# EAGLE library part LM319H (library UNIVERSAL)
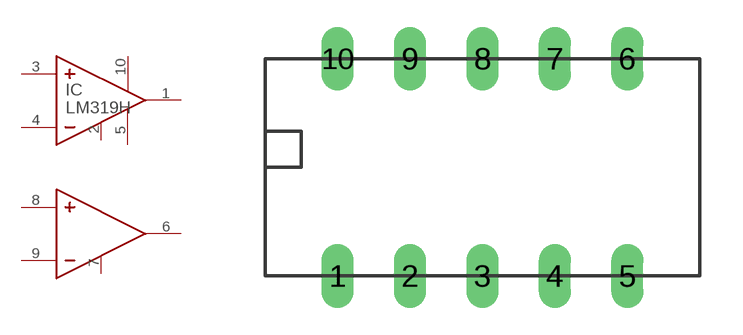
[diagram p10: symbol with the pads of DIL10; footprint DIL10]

Designator prefix IC

## LM319H  [DIL10]
1  1
2  2
3  3
4  4
5  5
6  6
7  7
8  8
9  9
10  10

## Footprint DIL10 (pad centres in mm)
drill 0.61 pad 1.092 long: 1 0,0; 2 2.54,0; 3 5.08,0; 4 7.62,0; 5 10.16,0; 6 10.16,7.62; 7 7.62,7.62; 8 5.08,7.62; 9 2.54,7.62; 10 0,7.62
